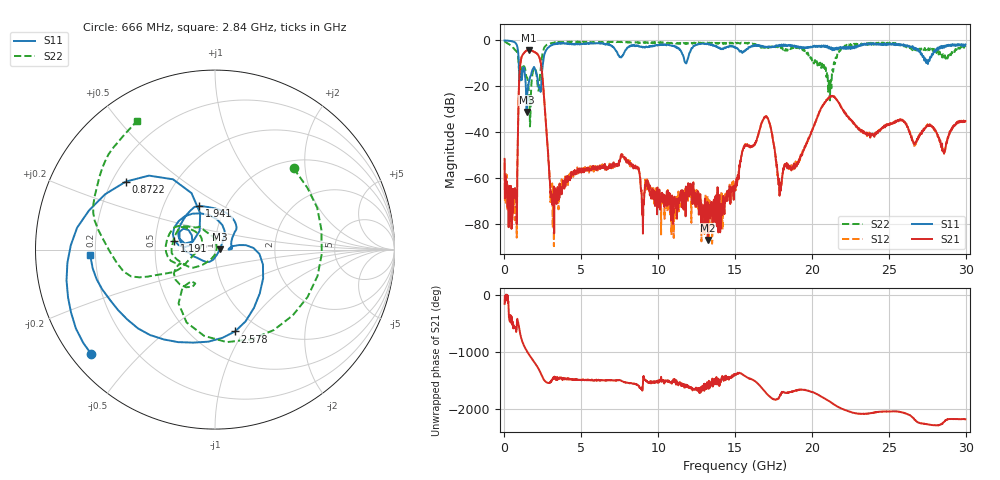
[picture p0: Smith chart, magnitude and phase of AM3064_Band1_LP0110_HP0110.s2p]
# Hz S DB R 50.0
!freq dBS11 angS11 dBS21 angS21 dBS12 angS12 dBS22 angS22
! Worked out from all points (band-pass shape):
!   1600 points, 10 MHz to 29.98 GHz, reference 50 ohm
!   highest |S21| = -4.20 dB at 1.584 GHz (marker M1); lowest = -87.0 dB at 13.22 GHz (marker M2)
!   |S21| within 3 dB of the highest: 1.119 GHz to 2.255 GHz (1.135 GHz wide, 67.3 % of centre)
!   lowest |S11| = -31.3 dB at 1.435 GHz (marker M3), VSWR 1.06, Z = 52.8 + j0.0908 ohm
!   |S11| at or under -10 dB: 931.6 MHz to 2.505 GHz (1.573 GHz wide, 91.6 % of centre); 11.8133 GHz to 11.82385 GHz (10.56 MHz wide, 0.0893 % of centre); 27.52404 GHz to 27.55143 GHz (27.39 MHz wide, 0.0995 % of centre)
!   |S22| runs from -37.5 to -0.4 dB; largest |S21 - S12| = 0.0094
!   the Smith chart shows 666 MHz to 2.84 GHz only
!   S11 on the Smith chart (normalised r, x): 666 MHz: 0.06, -0.36; 872.2 MHz: 0.26, +0.32; 1.191 GHz: 0.63, +0.07; 1.941 GHz: 0.75, +0.39; 2.578 GHz: 0.78, -0.92; 2.84 GHz: 0.18, -0.02
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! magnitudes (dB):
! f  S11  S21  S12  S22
! 10 MHz  0.0  -51.7  -53.3  -0.4
! 666 MHz  -0.9  -67.5  -78.4  -4.0
! 872.2 MHz  -4.1  -42.1  -42.0  -6.3
! 1.191 GHz  -12.7  -6.2  -6.1  -11.9
! 1.435 GHz  -31.3  -4.5  -4.4  -16.0
! 1.584 GHz  -18.3  -4.2  -4.2  -21.7
! 1.941 GHz  -11.8  -5.0  -5.0  -12.5
! 2.578 GHz  -6.6  -25.1  -25.2  -3.2
! 2.84 GHz  -3.1  -49.5  -49.2  -1.5
! 3.14 GHz  -1.9  -68.2  -81.7  -1.2
! 5.015 GHz  -1.5  -57.6  -56.5  -0.8
! 7.714 GHz  -6.4  -50.8  -50.4  -0.6
! 10 GHz  -2.0  -69.0  -67.7  -0.9
! 13.22 GHz  -1.4  -87.0  -71.4  -0.9
! 15 GHz  -3.0  -64.3  -62.9  -1.3
! 16.94 GHz  -2.9  -33.7  -33.3  -3.2
! 17.93 GHz  -2.0  -63.3  -62.3  -2.7
! 19.99 GHz  -3.1  -39.7  -39.6  -8.3
! 21.28 GHz  -3.6  -24.4  -24.4  -17.2
! 25 GHz  -1.4  -37.0  -36.6  -1.2
! 28.56 GHz  -2.6  -48.4  -48.5  -6.6
! 29.98 GHz  -1.8  -35.2  -35.3  -2.9
